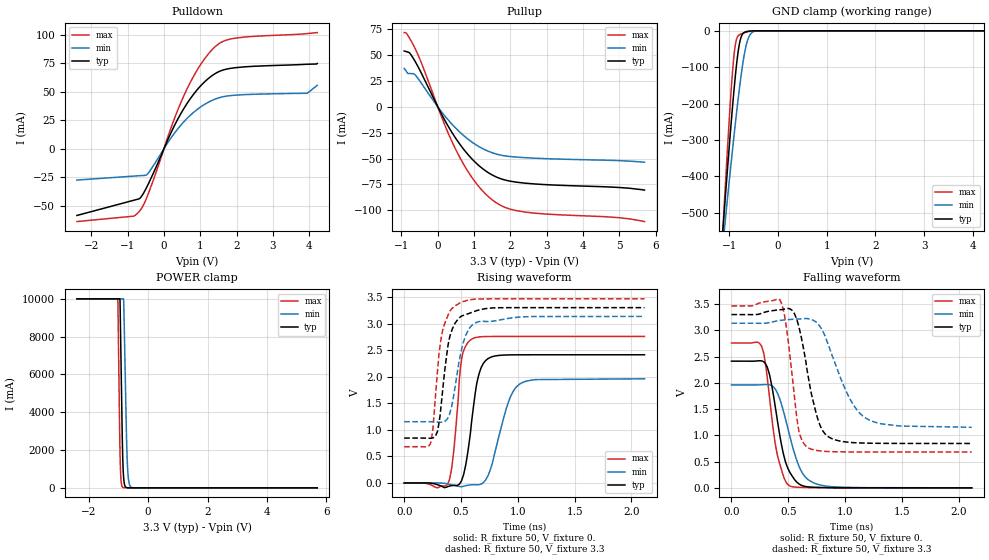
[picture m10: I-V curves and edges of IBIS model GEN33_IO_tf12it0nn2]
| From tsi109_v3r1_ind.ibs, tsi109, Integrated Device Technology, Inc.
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|   MODEL GEN33_IO_tf12it0nn2
[Model]   GEN33_IO_tf12it0nn2
Model_type  I/O
C_comp 1.247p 1.155p 1.342p
Polarity   Non-Inverting
Enable   Active-High
|   typ   min   max
Vinl   =   0.800v
Vinh   =   2.000v
Vmeas  =   1.65V
[Model Spec]
[Temperature Range]   25   125   -40
[Voltage Range] 3.3 3.135 3.465
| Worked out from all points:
|   slope of the pulldown table from 0 to 0.495 V, typ, clamps not added: 15.2 ohm
|   slope of the pullup table from 0 to 0.495 V, typ, clamps not added: 16.3 ohm
|   GND clamp passes 1 mA (typ) near -0.60 V on its own axis
|   POWER clamp passes 1 mA (typ) near -0.62 V on its own axis
|   rising waveform, R_fixture 50, V_fixture 0.: 20-80 % time 92.1ps typ, 147ps min, 63.9ps max; typ from 0 V to 2.41 V
|   rising waveform, R_fixture 50, V_fixture 3.3: 20-80 % time 90.2ps typ, 107ps min, 82.4ps max; typ from 0.845 V to 3.3 V
|   falling waveform, R_fixture 50, V_fixture 0.: 20-80 % time 121ps typ, 155ps min, 104ps max; typ from 2.41 V to 0 V
|   falling waveform, R_fixture 50, V_fixture 3.3: 20-80 % time 137ps typ, 233ps min, 88.9ps max; typ from 3.3 V to 0.845 V
[Pulldown]
-2.396V   -58.62mA   -27.49mA   -63.98mA
-836.4mV  -45.31mA   -24.03mA   -59.23mA
-662.3mV  -43.5mA    -23.65mA   -54.36mA
-555.2mV  -38.67mA   -23.41mA   -48.89mA
-441.4mV  -31.66mA   -21.77mA   -40.36mA
227.9mV   16.36mA    11.04mA    21.31mA
576mV     36.79mA    24.65mA    48.53mA
1.011V    55.29mA    36.77mA    74.07mA
1.46V     66.98mA    44.25mA    91.06mA
1.948V    71.23mA    47.09mA    97.19mA
3.95V     74.3mA     48.8mA     101.3mA
4.224V    74.99mA    55.83mA    102.2mA
[Pullup]
-924.1mV  53.85mA    37.04mA    71.64mA
-770.1mV  51.75mA    32.07mA    65.88mA
-656.3mV  45.76mA    31.75mA    58.52mA
-549.2mV  39.1mA     27.58mA    50.6mA
173.7mV   -11.72mA   -7.927mA   -15.86mA
588.7mV   -35.17mA   -23.83mA   -47.62mA
1.017V    -53.01mA   -35.88mA   -71.93mA
1.506V    -65.94mA   -44.44mA   -90.01mA
1.914V    -71.23mA   -47.69mA   -97.94mA
2.423V    -73.82mA   -49.19mA   -101.8mA
4.812V    -77.57mA   -51.77mA   -106.6mA
5.696V    -80.41mA   -53.59mA   -110.8mA
[GND Clamp]
-2.396V   -2.986A    -2.401A    -3.883A
-1.137V   -561.8mA   -599.1mA   -566.6mA
-1.105V   -504.5mA   -555.9mA   -489.3mA
-1.073V   -447.8mA   -513mA     -413.4mA
-977.8mV  -283.7mA   -386.7mA   -200.5mA
-914mV    -182.5mA   -305.4mA   -85.54mA
-858.3mV  -104.5mA   -237.1mA   -27.83mA
-786.5mV  -33.49mA   -155.3mA   -10.56mA
-730.8mV  -10.16mA   -99.42mA   -7.053mA
-643.1mV  -2.029mA   -35.61mA   -3.206mA
-475.8mV  -94.64uA   -1.218mA   -155.8uA
4.224V    0A         0A         0A
[Power Clamp]
-2.396V   10A        10A        10A
-1.024V   10A        10A        10A
-1.016V   10A        10A        9.745A
-944.9mV  9.88A      10A        1.741A
-913.3mV  6.804A     10A        429mA
-858.1mV  1.8A       10A        35.65mA
-818.7mV  442.1mA    9.697A     10.25mA
-732mV    17.95mA    3.021A     4.001mA
-700.4mV  6.514mA    1.351A     3.245mA
-653.1mV  1.962mA    364.6mA    2.275mA
-582.1mV  571.1uA    47.54mA    1.119mA
5.696V    0A         0A         0A
[Ramp]
dV/dt_r 1.448/92.129p 1.177/146.688p 1.655/63.888p
dV/dt_f 1.473/136.637p 1.19/233.06p 1.669/88.942p
[Rising Waveform]
R_fixture = 50
V_fixture = 0.
0s        514.3nV    829.9nV    0V
380ps     -72.22mV   -16.65mV   -30.18mV
435ps     -46.82mV   -40.63mV   580.9mV
505ps     46.06mV    -69.38mV   2.331V
595ps     1.188V     -33.37mV   2.708V
640ps     1.887V     -34.35mV   2.742V
700ps     2.26V      13.25mV    2.755V
915ps     2.41V      1.509V     2.758V
1.015ns   2.412V     1.858V     2.758V
2.115ns   2.413V     1.961V     2.758V
[Rising Waveform]
R_fixture = 50
V_fixture = 3.3
V_fixture_min = 3.135
V_fixture_max = 3.465
0s        845.1mV    1.152V     682.8mV
230ps     841.1mV    1.152V     737.3mV
250ps     847mV      1.151V     968.8mV
290ps     953.2mV    1.146V     2.027V
325ps     1.463V     1.144V     2.721V
390ps     2.643V     1.25V      3.179V
485ps     3.108V     2.305V     3.382V
560ps     3.183V     2.862V     3.439V
660ps     3.256V     3.038V     3.463V
2.115ns   3.3V       3.135V     3.465V
[Falling Waveform]
R_fixture = 50
V_fixture = 0.
0s        2.413V     1.961V     2.758V
265ps     2.417V     1.963V     2.699V
290ps     2.388V     1.966V     2.493V
335ps     2.157V     1.962V     1.726V
405ps     1.275V     1.803V     617.3mV
455ps     667mV      1.481V     243.1mV
505ps     334.2mV    1.06V      47.32mV
610ps     55.17mV    338.4mV    9.261mV
750ps     9.81mV     73.13mV    2.4mV
2.115ns   27.36uV    31.28uV    27.88uV
[Falling Waveform]
R_fixture = 50
V_fixture = 3.3
V_fixture_min = 3.135
V_fixture_max = 3.465
0s        3.3V       3.135V     3.465V
430ps     3.392V     3.189V     3.563V
485ps     3.413V     3.201V     3.039V
595ps     3.058V     3.216V     1.074V
680ps     2.068V     3.219V     758mV
760ps     1.311V     3.126V     708.7mV
825ps     1.025V     2.886V     694.2mV
1.025ns   869.6mV    1.77V      684.3mV
1.185ns   851.7mV    1.324V     683.2mV
2.115ns   845.2mV    1.153V     682.9mV
